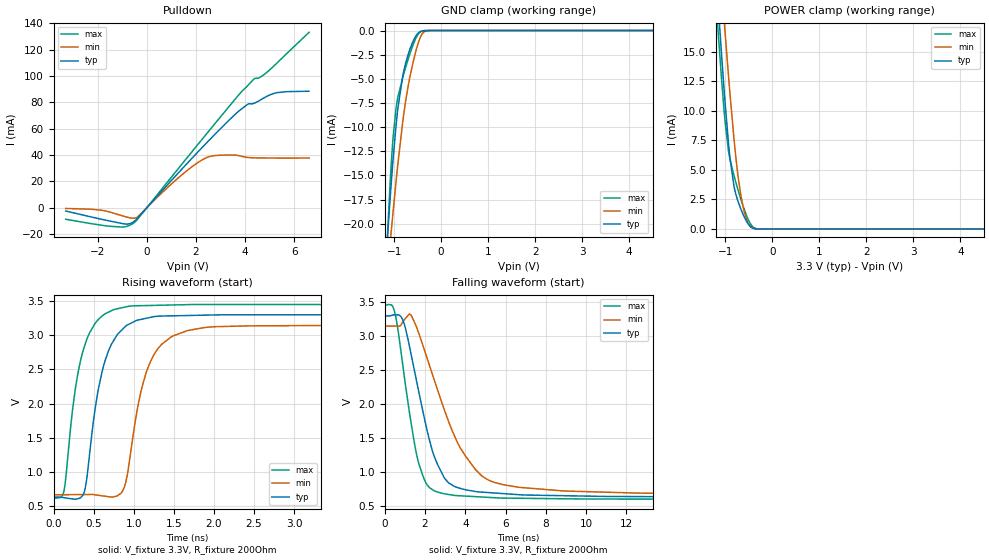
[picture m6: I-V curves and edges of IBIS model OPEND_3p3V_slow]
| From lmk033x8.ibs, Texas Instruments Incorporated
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[Model]   OPEND_3p3V_slow
Model_type   Open_drain
Polarity   Non-Inverting
Vmeas = 1.65
Vref = 3.3
Cref = 15pF
Rref = 200
|   typ   min   max
|   (nom PVT)   (fast PVT)   (slow PVT)
C_comp   0.571p   0.551p   0.636p
|C_comp (ON state)   0.733p   0.694p   0.771p
|C_comp (OFF state)   0.571p   0.551p   0.636p
[Voltage Range]   3.3   3.15   3.45
[Temperature Range]   27   125   -40
[Pullup Reference]   3.3   3.15   3.45
[Pulldown Reference]   0   0   0
[Power Clamp Reference]   3.3   3.15   3.45
[GND Clamp Reference]   0   0   0
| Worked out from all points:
|   slope of the pulldown table from 0 to 0.495 V, typ, clamps not added: 48 ohm
|   GND clamp passes 1 mA (typ) near -0.58 V on its own axis
|   POWER clamp passes 1 mA (typ) near -0.60 V on its own axis
|   falling waveform, V_fixture 3.3V, R_fixture 200Ohm: 20-80 % time 1.26ns typ, 2.05ns min, 894ps max; typ from 3.3 V to 0.632 V
|   rising waveform, V_fixture 3.3V, R_fixture 200Ohm: 20-80 % time 244ps typ, 278ps min, 223ps max; typ from 0.63 V to 3.3 V
[Pulldown]
|   Voltage   I(typ)   I(min)   I(max)
-3.3V     -2.52mA    -600.3uA   -8.758mA
-1.865V   -8.706mA   -1.855mA   -13.25mA
-963.6mV  -12.15mA   -6.33mA    -14.77mA
-528mV    -10.55mA   -7.967mA   -11.61mA
-379.5mV  -7.92mA    -6.939mA   -8.819mA
1.541V    31.66mA    26.77mA    35.73mA
2.511V    50.79mA    38.65mA    57.96mA
3.482V    68.92mA    40.03mA    79.92mA
4.125V    78.74mA    38.11mA    93.15mA
4.372V    79.36mA    37.88mA    97.98mA
5.273V    87.34mA    37.74mA    109.6mA
6.6V      88.5mA     37.75mA    133.2mA
[GND Clamp]
|   Voltage   I(typ)   I(min)   I(max)
-3.3V     -203.8mA   -156.3mA   -307mA
-1.171V   -23.41mA   -26.67mA   -23.99mA
-1.073V   -16.48mA   -21.32mA   -14.64mA
-1.053V   -15.2mA    -20.29mA   -13.1mA
-1.023V   -13.35mA   -18.76mA   -11.08mA
-963.6mV  -10.02mA   -15.81mA   -8.174mA
-924mV    -8.154mA   -13.94mA   -6.971mA
-815.1mV  -4.636mA   -9.357mA   -4.815mA
-636.9mV  -1.582mA   -4.164mA   -2.006mA
-438.9mV  -95.08uA   -660.3uA   -145.6uA
-260.7mV  -658.8nA   -9.216uA   -902.5nA
6.6V      0A         0A         0A
[POWER Clamp]
|   Voltage   I(typ)   I(min)   I(max)
-3.3V     163.1mA    154.7mA    175.2mA
-1.162V   19.42mA    25.01mA    17.09mA
-1.092V   15.36mA    21.2mA     13.24mA
-1.013V   11.02mA    16.97mA    9.368mA
-933.9mV  7.229mA    12.94mA    6.584mA
-904.2mV  6.039mA    11.5mA     5.927mA
-815.1mV  3.558mA    7.522mA    4.491mA
-716.1mV  2.165mA    4.038mA    3.108mA
-656.7mV  1.543mA    2.548mA    2.342mA
-567.6mV  770.8uA    1.019mA    1.318mA
-409.2mV  60.75uA    64.51uA    154.9uA
6.6V      0A         0A         0A
[Ramp]
R_load = 200
|   typ   min   max
dV/dt_r   1.60172/2.43354e-10   1.49099/2.76451e-10   1.70398/2.22645e-10
dV/dt_f   1.60078/1.25929e-09   1.48593/2.04304e-09   1.70973/8.9342e-10
[Falling Waveform]
V_fixture = 3.3V
V_fixture_min = 3.15V
V_fixture_max = 3.45V
R_fixture = 200Ohm
C_fixture = 0F
|   Time   V(typ)   V(min)   V(max)
0s        3.3V       3.15V      3.449V
493.9ps   3.314V     3.149V     3.354V
922ps     3.221V     3.226V     2.514V
1.253ns   2.813V     3.326V     1.825V
1.664ns   2.219V     3.065V     1.154V
2.439ns   1.246V     2.373V     728.3mV
2.985ns   903.8mV    1.895V     679.3mV
3.779ns   758.1mV    1.342V     650.8mV
5.369ns   694.1mV    856.6mV    624.3mV
19ns      632mV      673.5mV    599.2mV
[Rising Waveform]
V_fixture = 3.3V
V_fixture_min = 3.15V
V_fixture_max = 3.45V
R_fixture = 200Ohm
C_fixture = 0F
|   Time   V(typ)   V(min)   V(max)
0s        630.5mV    665mV      610mV
129ps     623.3mV    666.3mV    713.1mV
269.2ps   599.1mV    667.7mV    2.192V
413.9ps   893.6mV    669.2mV    2.937V
628ps     2.568V     646.7mV    3.301V
933.8ps   3.158V     1.055V     3.423V
1.091ns   3.232V     2.177V     3.433V
1.244ns   3.27V      2.698V     3.437V
1.886ns   3.294V     3.113V     3.45V
19ns      3.3V       3.15V      3.45V
